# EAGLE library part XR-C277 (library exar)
Low voltage REPEATER
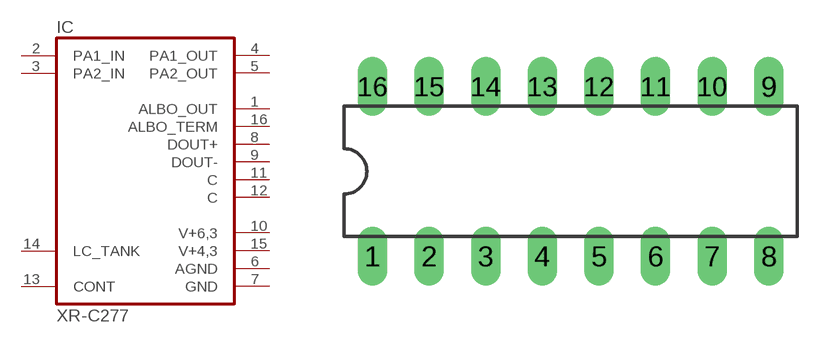
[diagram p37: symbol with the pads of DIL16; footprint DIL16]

Designator prefix IC

## XR-C277 (OC_FARNELL: unknown; OC_NEWARK: unknown)  [DIL16]
1  ALBO_OUT  out
2  PA1_IN  in
3  PA2_IN  in
4  PA1_OUT  out
5  PA2_OUT  out
6  AGND  pwr
7  GND  pwr
8  DOUT+  out
9  DOUT-  out
10  V+6,3  pwr
11  C  out
12  C  out
13  CONT  pas
14  LC_TANK  in
15  V+4,3  pwr
16  ALBO_TERM  out

## Footprint DIL16 (pad centres in mm)
Dual In Line Package
drill 0.813 long: 1 -8.89,-3.81; 2 -6.35,-3.81; 3 -3.81,-3.81; 4 -1.27,-3.81; 5 1.27,-3.81; 6 3.81,-3.81; 7 6.35,-3.81; 8 8.89,-3.81; 9 8.89,3.81; 10 6.35,3.81; 11 3.81,3.81; 12 1.27,3.81; 13 -1.27,3.81; 14 -3.81,3.81; 15 -6.35,3.81; 16 -8.89,3.81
